FUNCTION_BLOCK "Main"
VERSION : 0.1
   VAR_TEMP
      temp1 : Bool;
      temp2 : Bool;
   END_VAR
BEGIN
NETWORK
TITLE =
      SET;
      = temp1;
      = temp2;
      JU lab0;
      CALL "__CPROVER_assert"
      (  condition := FALSE
      );
lab0: SET;
lab1: A temp1;
      A temp2;
      NOT;
      = temp2;
      A temp2;

      JCN lab1;
      CALL "__CPROVER_assert"
      (  condition := #temp2
      );

      JC lab2;
      CALL "__CPROVER_assert"
      (  condition := FALSE
      );

lab2: NOP 0;

END_FUNCTION_BLOCK

